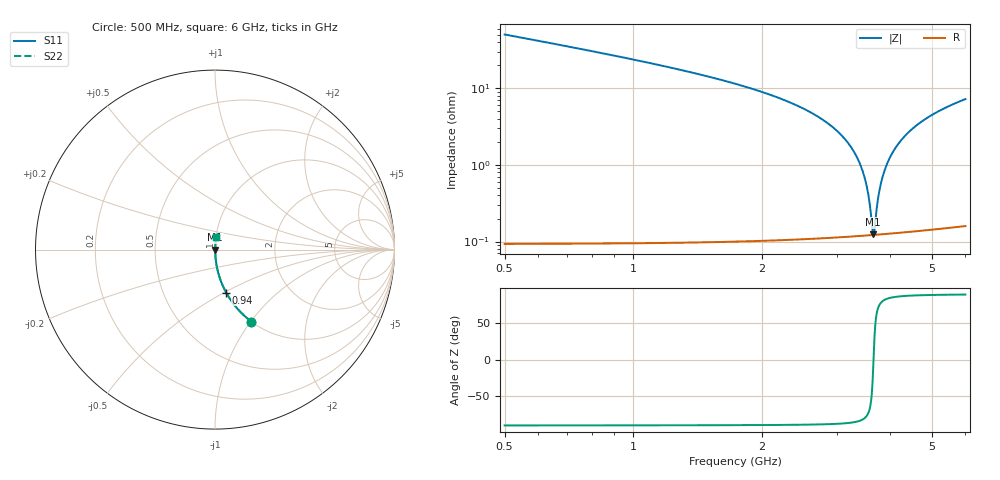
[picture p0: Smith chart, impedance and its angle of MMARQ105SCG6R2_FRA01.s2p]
! MMARQ105SCG6R2_FRA01  S-PARAMETER MODEL  ( General Type )
! Model Generated by TAIYO YUDEN Corporation (http://www.ty-top.com)
! Version 1.0
! TAIYO YUDEN Control No. 200326
! Copyright(c) 2020 TAIYO YUDEN CO.,LTD. All Rights Reserved.
! Product Description (link to TY-COMPAS)
! https://ds.yuden.co.jp/TYCOMPAS/or/detail?pn=MMARQ105SCG6R2CFRA01&u=M
! Products Name : Multilayer Ceramic Capacitors
! Characteristics :
!  Capacitance : 6.2 pF , Rated Voltage : 250V , TCC : CG / C0G
!  Case Size : 1.0 x 0.5 / 0.039 x 0.02 [mm/inch] , Thickness : 0.5 / 0.02 [mm/inch]
!  (Conditions: Temperature = 25 degC , DC Bias Current/Voltage = 0A / 0V)
! External Node Assignments :
!  1  o---| |---o  2
! GND o---------o GND
! Frequency Range : 500MHz  -  6GHz  [ 401 STEP ]
# MHz S RI R 50
! Freq[MHz].  S11 Real  S11 Imag  S21 Real  S21 Imag  S12 Real  S12 Imag  S22 Real  S22 Imag
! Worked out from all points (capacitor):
!   401 points, 500 MHz to 6 GHz, reference 50 ohm
!   read as one part in series: C = 6.2 pF near 527.5 MHz
!   lowest |Z| = 125 mohm at 3.649 GHz (marker M1)
!   series resonance near 3.656 GHz, so ESL is about 310 pH
!   S11 on the Smith chart (normalised r, x): 500 MHz: 1.00, -1.01; 940 MHz: 1.00, -0.51; 6 GHz: 1.00, +0.14
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500  0.2029 -0.4012  0.7971 0.4012  0.7971 0.4012  0.2029 -0.4012
692.5  0.1139 -0.3164  0.8861 0.3164  0.8861 0.3164  0.1139 -0.3164
940  0.0619 -0.239  0.9381 0.239  0.9381 0.239  0.0619 -0.239
1421.25  0.0239 -0.1495  0.9761 0.1495  0.9761 0.1495  0.0239 -0.1495
2342.5  0.00519 -0.0642  0.9948 0.0642  0.9948 0.0642  0.00519 -0.0642
2892.5  0.00221 -0.033  0.9978 0.033  0.9978 0.033  0.00221 -0.033
3085  0.00171 -0.0239  0.9983 0.0239  0.9983 0.0239  0.00171 -0.0239
3250  0.00144 -0.0165  0.9986 0.0165  0.9986 0.0165  0.00144 -0.0165
3387.5  0.0013 -0.0107  0.9987 0.0107  0.9987 0.0107  0.0013 -0.0107
3497.5  0.00123 -0.00619  0.9988 0.00619  0.9988 0.00619  0.00123 -0.00619
3566.25  0.00122 -0.00346  0.9988 0.00346  0.9988 0.00346  0.00122 -0.00346
3621.25  0.00122 -0.00132  0.9988 0.00132  0.9988 0.00132  0.00122 -0.00132
3648.75  0.00122 -0.000261  0.9988 0.000261  0.9988 0.000261  0.00122 -0.000261
3676.25  0.00122 0.000789  0.9988 -0.000789  0.9988 -0.000789  0.00122 0.000789
3731.25  0.00124 0.00287  0.9988 -0.00287  0.9988 -0.00287  0.00124 0.00287
3772.5  0.00125 0.00441  0.9987 -0.00441  0.9987 -0.00441  0.00125 0.00441
3855  0.0013 0.00743  0.9987 -0.00743  0.9987 -0.00743  0.0013 0.00743
3992.5  0.00142 0.0123  0.9986 -0.0123  0.9986 -0.0123  0.00142 0.0123
4171.25  0.00164 0.0185  0.9984 -0.0185  0.9984 -0.0185  0.00164 0.0185
4556.25  0.00232 0.031  0.9977 -0.031  0.9977 -0.031  0.00232 0.031
5092.5  0.00366 0.0471  0.9963 -0.0471  0.9963 -0.0471  0.00366 0.0471
6000  0.00676 0.0717  0.9932 -0.0717  0.9932 -0.0717  0.00676 0.0717
